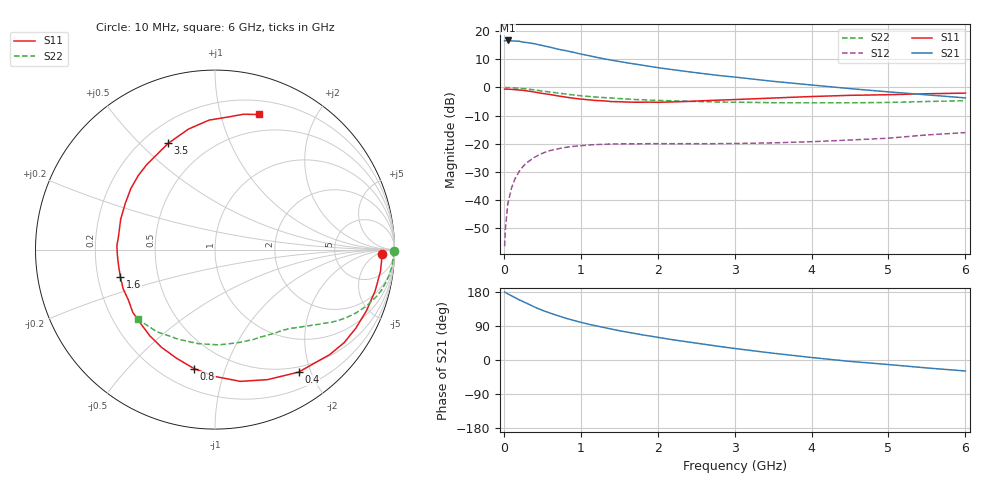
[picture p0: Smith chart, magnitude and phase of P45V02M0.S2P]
! SIEMENS Small Signal Semiconductors
! BFP182
! Si NPN RF Bipolar Junction Transistor in SOT143
! VCE = 5 V  IC = 2 mA
! Common Emitter S-Parameters:  March  1996
# GHz  S  MA  R  50
!  f  S11  S21  S12  S22
! GHz  MAG  ANG  MAG  ANG  MAG  ANG  MAG  ANG
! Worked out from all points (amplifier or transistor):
!   36 points, 10 MHz to 6 GHz, reference 50 ohm
!   highest |S21| = 16.7 dB at 50 MHz (marker M1)
!   |S21| within 3 dB of that: start of sweep to 687.5 MHz
!   unconditionally stable (mu >= 1): 2.228 GHz to 5.906 GHz
!   at 250 MHz: K = 0.12, MSG = 22.1 dB, |S12| = -28.1 dB
!   at 1.4 GHz: K = 0.66, MSG = 14.9 dB, |S12| = -20.1 dB
!   at 6 GHz: K = 0.98, MSG = 6.2 dB, |S12| = -16.1 dB
!   lowest NFmin = 1.10 dB at 450 MHz
!   S11 on the Smith chart (normalised r, x): 10 MHz: 25, -9; 400 MHz: 0.42, -1.82; 800 MHz: 0.32, -0.79; 1.6 GHz: 0.30, -0.13; 3.5 GHz: 0.30, +0.61; 6 GHz: 0.33, +1.32
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0.01  0.9318 -1.4  6.735 179.2  0.0015 84.2  0.9954 -0.5
0.02  0.9309 -2.8  6.753 178.4  0.003 90.7  0.9899 -1.1
0.05  0.9299 -7.4  6.833 174.6  0.0083 88.3  0.9937 -2.8
0.1  0.9216 -14.4  6.713 169.4  0.0163 81.3  0.9893 -5.7
0.2  0.8985 -29.2  6.613 158.8  0.032 73.2  0.9682 -11.1
0.4  0.8263 -55.7  5.976 139.7  0.0573 58.5  0.9008 -20.4
0.5  0.7814 -68.0  5.551 131.2  0.0674 51.9  0.8621 -24.1
0.6  0.7477 -79.1  5.189 124.0  0.0752 46.8  0.8274 -27.1
0.7  0.7066 -90.1  4.789 117.1  0.0806 42.0  0.7937 -29.8
0.8  0.6731 -100.0  4.513 110.7  0.0855 37.8  0.763 -32.1
0.9  0.6422 -109.5  4.217 104.9  0.0895 34.4  0.7336 -34.0
1.1  0.6018 -127.2  3.679 94.5  0.0943 28.4  0.6896 -37.5
1.3  0.5766 -142.6  3.231 85.8  0.0973 23.8  0.6581 -40.4
1.5  0.5563 -157.0  2.89 77.3  0.0988 20.8  0.6327 -43.2
1.6  0.5487 -163.9  2.738 73.7  0.0995 19.2  0.6224 -44.5
1.8  0.5447 -176.8  2.483 66.4  0.0995 17.6  0.6018 -47.1
2.2  0.5522 162.1  2.061 53.3  0.0997 14.7  0.5773 -52.9
2.8  0.594 136.1  1.626 35.8  0.1 13.7  0.5487 -62.7
3.5  0.6468 113.8  1.282 17.9  0.1032 14.6  0.5341 -76.5
4.5  0.7223 92.6  0.951 -3.7  0.1158 17.3  0.5323 -100.0
5.5  0.7702 78.2  0.736 -21.0  0.1428 18.0  0.561 -125.5
6  0.7918 72.0  0.65 -29.0  0.1569 15.0  0.5793 -138.1
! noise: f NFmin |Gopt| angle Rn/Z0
0.45  1.1  0.42  29  0.36
0.9  1.2  0.4  58  0.3
1.8  1.85  0.32  126  0.22
